PROGRAM MAIN
VAR
	fbClient:FB_IotHttpClient:=(sHostName:='127.0.0.1',bKeepAlive:=TRUE,	tConnectionTimeout:=T#10S);
	fbGetProductByBarCode:FB_GetProductByBarCode;
	fbGetPagedProducts:FB_GetPagedProducts;
	fbAddProduct:FB_AddProduct;
	fbDeleteProductById:FB_DeleteProductById;
	fbUpdateProduc:FB_UpdateProduct;
END_VAR

IF NOT fbClient.bConfigured THEN 
	fbClient.nHostPort:= 5000;
	fbClient.stTLS.bNoServerCertCheck:= FALSE;
END_IF

fbClient.Execute();

fbGetProductByBarCode(fbClient:=fbClient , bBusy=> , bError=>);

fbGetPagedProducts(fbClient:=fbClient , bBusy=> , bError=> );
fbAddProduct(fbClient:=fbClient , bBusy=> , bError=> );
fbDeleteProductById(fbClient:=fbClient , bBusy=> , bError=> );
fbUpdateProduc(fbClient:=fbClient , bBusy=> , bError=> );

END_PROGRAM
